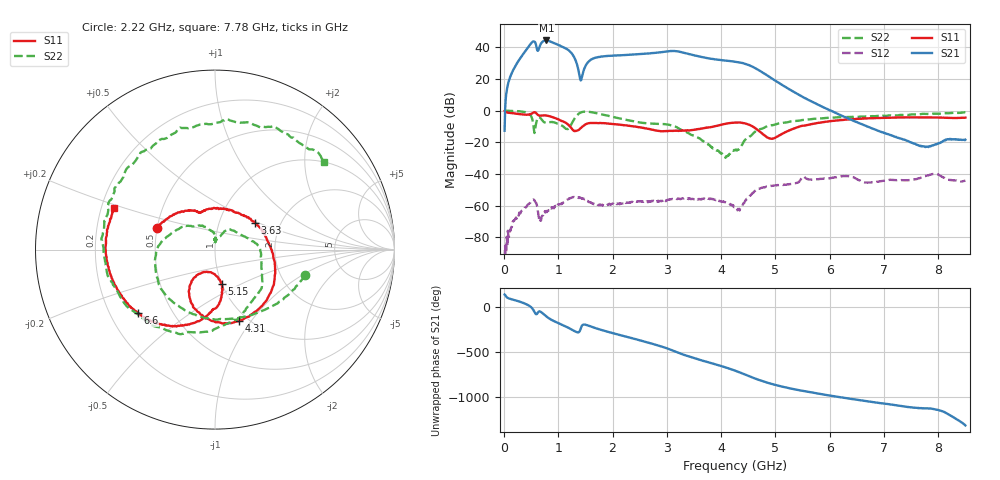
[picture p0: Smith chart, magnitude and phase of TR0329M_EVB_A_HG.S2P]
!Agilent Technologies,E5071C,MY46523237,B.13.01
!Date: Thu Mar 10 13:22:39 2022
!Data & Calibration Information:
!Freq	S11:SOLT2(ON)	S21:SOLT2(ON)	S12:SOLT2(ON)	S22:SOLT2(ON)
!PortZ  Port1:50+j0  Port2:50+j0
!Above PortZ is port z conversion or system Z0 setting when saving the data.
!When reading, reference impedance value at option line is always used.
# Hz S dB R 50
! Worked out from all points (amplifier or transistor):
!   850 points, 10 MHz to 8.5 GHz, reference 50 ohm
!   highest |S21| = 44.3 dB at 780 MHz (marker M1)
!   |S21| within 3 dB of that: 665.6 MHz to 1.012 GHz (346.3 MHz wide, 41.3 % of centre)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
!   unconditionally stable (mu >= 1): 24.8 MHz to 172.1 MHz; 577.4 MHz to 1.519 GHz; 1.521 GHz to end of sweep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
!   at 1.42 GHz: K = 6.47, MAG = 26.2 dB, |S12| = -55.4 dB
!   at 4.26 GHz: K = 13.24, MAG = 31.7 dB, |S12| = -61.0 dB
!   at 8.5 GHz: K = 103.24, MAG = -10.2 dB, |S12| = -44.3 dB
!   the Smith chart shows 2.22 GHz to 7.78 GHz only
!   S11 on the Smith chart (normalised r, x): 2.22 GHz: 0.50, +0.14; 3.63 GHz: 1.48, +0.48; 4.31 GHz: 0.90, -0.88; 5.15 GHz: 1.00, -0.40; 6.6 GHz: 0.32, -0.32; 7.78 GHz: 0.25, +0.19
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1e7  -0.24 -4.6  -12.77 140.4  -93.64 -166.6  -0.01 -73.0
3.9e8  -2.61 -47.4  37.45 37.6  -61.27 57.3  -0.96 130.1
5.1e8  -1.91 -57.0  43.01 -7.3  -56.84 17.5  -4.42 93.9
5.7e8  -1.13 -75.9  43.31 -64.2  -57.44 -24.3  -12.66 143.1
6.9e8  -3.19 -86.9  42.78 -59.0  -67.31 5.2  -5.55 113.6
7.8e8  -3.14 -100.1  44.30 -105.4  -63.43 1.6  -7.73 117.3
9.2e8  -4.49 -121.0  42.65 -156.6  -61.74 -10.0  -7.42 113.5
1.14e9  -7.84 -146.4  39.22 142.8  -56.87 -46.5  -11.53 118.3
1.43e9  -10.56 -121.2  20.43 148.6  -55.35 -161.3  -0.99 112.8
1.65e9  -7.88 -147.5  32.96 132.4  -59.21 111.4  -1.29 64.6
2.22e9  -9.25 159.6  35.07 34.7  -58.63 21.9  -5.64 -15.8
2.84e9  -12.91 113.6  36.63 -69.2  -56.94 -27.7  -8.46 -114.7
3.23e9  -12.76 83.4  37.16 -154.6  -55.72 -51.6  -11.55 161.7
3.63e9  -11.39 33.8  33.92 126.4  -56.09 -75.5  -18.31 107.3
4.26e9  -7.56 -63.0  30.83 9.1  -60.97 -96.4  -25.08 93.6
4.31e9  -7.52 -71.5  30.61 -1.8  -62.09 -79.5  -24.69 87.7
5.15e9  -14.22 -79.0  15.64 -172.1  -46.95 -129.8  -7.73 -77.1
5.67e9  -8.53 -97.6  5.67 126.0  -43.70 176.9  -5.35 -127.2
6.6e9  -5.09 -140.8  -8.75 35.9  -44.94 72.1  -3.78 155.2
7.09e9  -4.51 -163.5  -15.09 -5.4  -43.87 47.7  -3.05 106.6
7.78e9  -4.34 157.6  -22.91 -52.5  -41.24 -10.9  -2.13 38.8
8.5e9  -4.49 110.0  -18.42 117.6  -44.25 -117.8  -1.17 -14.2
